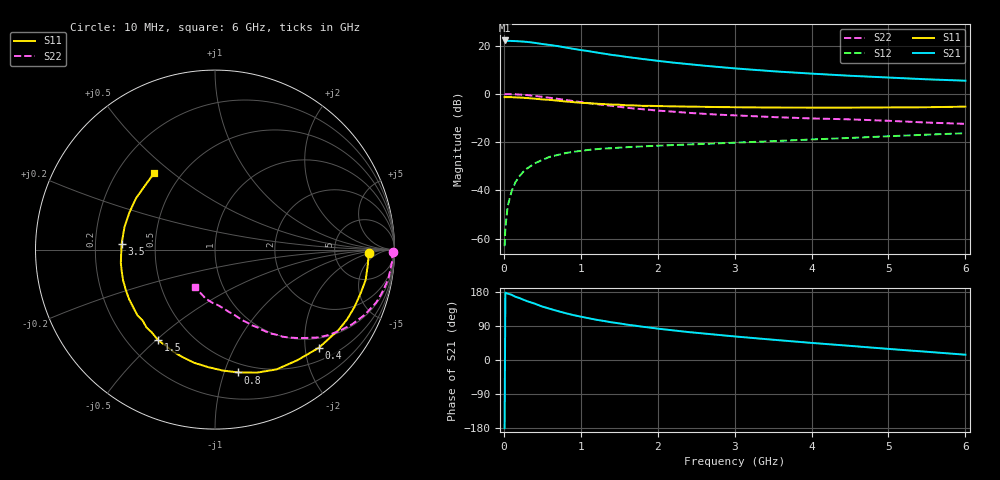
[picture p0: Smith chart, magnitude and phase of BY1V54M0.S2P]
! SIEMENS Small Signal Semiconductors
! BFY420
! Si NPN RF SIEGET Grounded Emitter Transistor in MICRO-X
! VCE = 1.5 V  IC = 4 mA
! Common Emitter S-Parameters:  October  1996
# GHz  S  MA  R  50
!  f  S11  S21  S12  S22
! GHz  MAG  ANG  MAG  ANG  MAG  ANG  MAG  ANG
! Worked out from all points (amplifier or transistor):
!   36 points, 10 MHz to 6 GHz, reference 50 ohm
!   highest |S21| = 22.1 dB at 10 MHz (marker M1)
!   |S21| within 3 dB of that: start of sweep to 817.2 MHz
!   unconditionally stable (mu >= 1): 3.324 GHz to end of sweep
!   at 250 MHz: K = 0.09, MSG = 27.0 dB, |S12| = -32.4 dB
!   at 1.4 GHz: K = 0.47, MSG = 19.3 dB, |S12| = -22.5 dB
!   at 6 GHz: K = 1.17, MAG = 8.4 dB, |S12| = -16.3 dB
!   S11 on the Smith chart (normalised r, x): 10 MHz: 13, -2; 400 MHz: 0.77, -2.29; 800 MHz: 0.42, -1.12; 1.5 GHz: 0.32, -0.51; 3.5 GHz: 0.31, +0.03; 6 GHz: 0.36, +0.43
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0.01  0.8567 -1.3  12.8 -180.0  0.0007 99.2  0.9914 -0.7
0.02  0.8558 -2.4  12.77 177.9  0.0017 106.6  0.9837 -1.1
0.05  0.8557 -5.6  12.54 175.1  0.0047 88.0  0.9909 -3.1
0.1  0.8562 -11.4  12.51 172.1  0.0095 83.5  0.9839 -6.2
0.15  0.8472 -16.6  12.41 166.9  0.0147 80.9  0.9799 -9.4
0.25  0.8325 -27.8  12.14 159.4  0.0241 74.8  0.9576 -15.3
0.3  0.8214 -33.0  11.94 155.4  0.0283 72.1  0.9451 -18.2
0.4  0.7961 -43.4  11.45 148.8  0.0363 67.2  0.9093 -23.6
0.5  0.7685 -53.3  10.8 141.0  0.043 62.1  0.8704 -28.5
0.6  0.7505 -62.8  10.32 135.1  0.0498 57.9  0.83 -33.0
0.8  0.6964 -79.3  9.166 123.7  0.0593 50.2  0.7495 -40.8
0.9  0.6753 -86.3  8.589 118.7  0.063 47.6  0.711 -43.8
1.1  0.6414 -100.3  7.697 110.3  0.0691 42.7  0.6451 -49.5
1.3  0.6147 -112.0  6.83 103.0  0.074 39.1  0.5882 -53.9
1.5  0.5963 -122.0  6.153 96.7  0.0769 36.2  0.5397 -58.0
1.8  0.5647 -135.5  5.288 87.9  0.0816 33.6  0.4823 -62.5
2.2  0.5525 -150.1  4.451 78.2  0.0871 30.9  0.429 -68.0
2.8  0.5333 -167.2  3.604 66.0  0.0948 28.6  0.3703 -74.8
3.5  0.5214 176.6  2.946 53.5  0.1051 27.0  0.3313 -81.8
4.5  0.5199 156.2  2.375 37.3  0.1224 23.5  0.2968 -92.8
5.5  0.5294 136.8  2.005 21.7  0.1431 19.0  0.2549 -108.5
6  0.5446 128.5  1.878 14.0  0.1534 15.8  0.2396 -118.3
